(* Logix 5000 AddOnInstructionDefinition export Banner_RSio_Reset_v1; software revision 33.00 *)

TYPE Banner_RSio_Reset_Main_v1 :
STRUCT
   Reset_Ownership : BOOL;
   Array1 : SINT[30];
   Array2 : SINT[30];
END_STRUCT
END_TYPE

ADD_ON_INSTRUCTION Banner_RSio_Reset_v1   (* revision 1.0 *)
VAR_IN_OUT
   Read : MESSAGE; {required}
   Write : MESSAGE; {required}
   RSio : Banner_RSio_Reset_Main_v1; {required}
END_VAR
VAR_OUTPUT
   Busy : BOOL; {visible}
   Done : BOOL; {visible}
   Error : BOOL; {visible}
   Error_Code : DINT; {access Read Only, visible}
END_VAR
VAR
   Timer2 : TIMER := (PRE := 20000); {access None}
   Timer1 : TIMER := (PRE := 20000); {access None}
   ConReset : DINT; {access None}
END_VAR

ROUTINE Logic   (* ladder *)
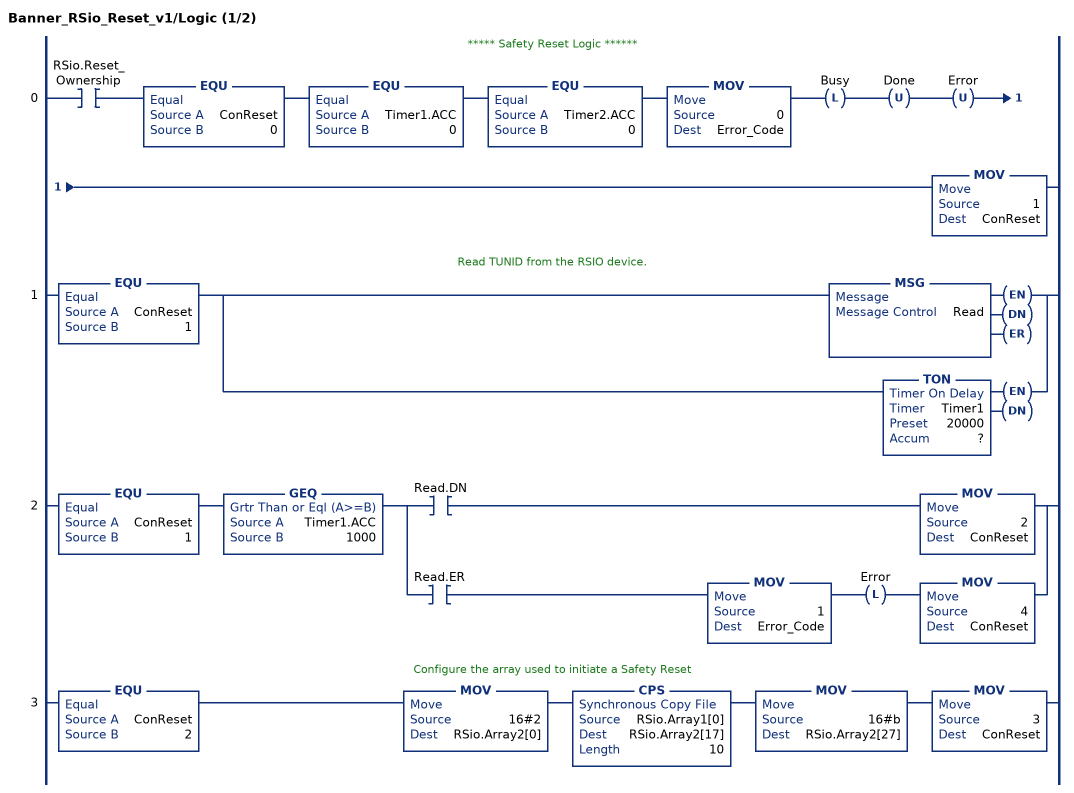
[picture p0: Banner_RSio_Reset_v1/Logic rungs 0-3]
   // ***** Safety Reset Logic ******
   0: XIC(RSio.Reset_Ownership)EQU(ConReset,0)EQU(Timer1.ACC,0)EQU(Timer2.ACC,0)MOV(0,Error_Code)OTL(Busy)OTU(Done)OTU(Error)MOV(1,ConReset);
   // Read TUNID from the RSIO device.
   1: EQU(ConReset,1)[MSG(Read) ,TON(Timer1,?,?) ];
   2: EQU(ConReset,1)GEQ(Timer1.ACC,1000)[XIC(Read.DN) MOV(2,ConReset) ,XIC(Read.ER) MOV(1,Error_Code) OTL(Error) MOV(4,ConReset) ];
   // Configure the array used to initiate a Safety Reset
   3: EQU(ConReset,2)MOV(16#2,RSio.Array2[0])CPS(RSio.Array1[0],RSio.Array2[17],10)MOV(16#b,RSio.Array2[27])MOV(3,ConReset);
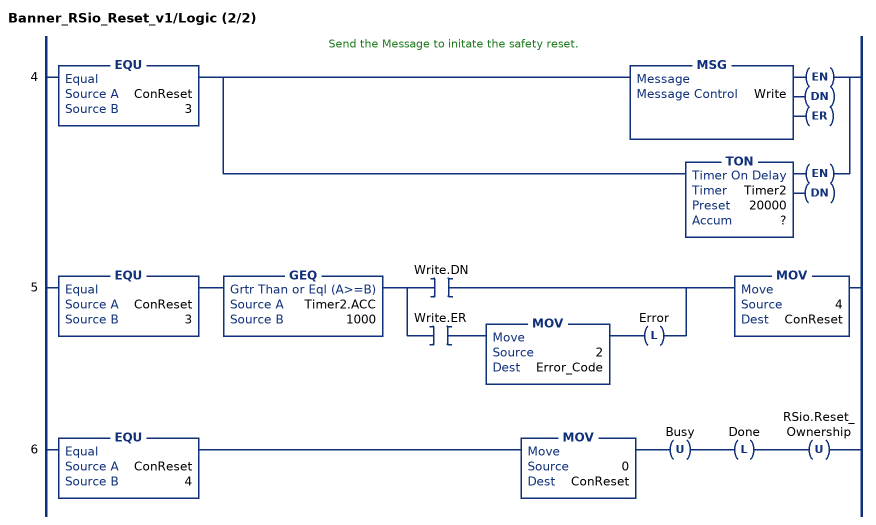
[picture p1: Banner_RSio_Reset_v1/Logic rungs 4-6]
   // Send the Message to initate the safety reset.
   4: EQU(ConReset,3)[MSG(Write) ,TON(Timer2,?,?) ];
   5: EQU(ConReset,3)GEQ(Timer2.ACC,1000)[XIC(Write.DN) ,XIC(Write.ER) MOV(2,Error_Code) OTL(Error) ]MOV(4,ConReset);
   6: EQU(ConReset,4)MOV(0,ConReset)OTU(Busy)OTL(Done)OTU(RSio.Reset_Ownership);
END_ROUTINE
END_ADD_ON_INSTRUCTION
